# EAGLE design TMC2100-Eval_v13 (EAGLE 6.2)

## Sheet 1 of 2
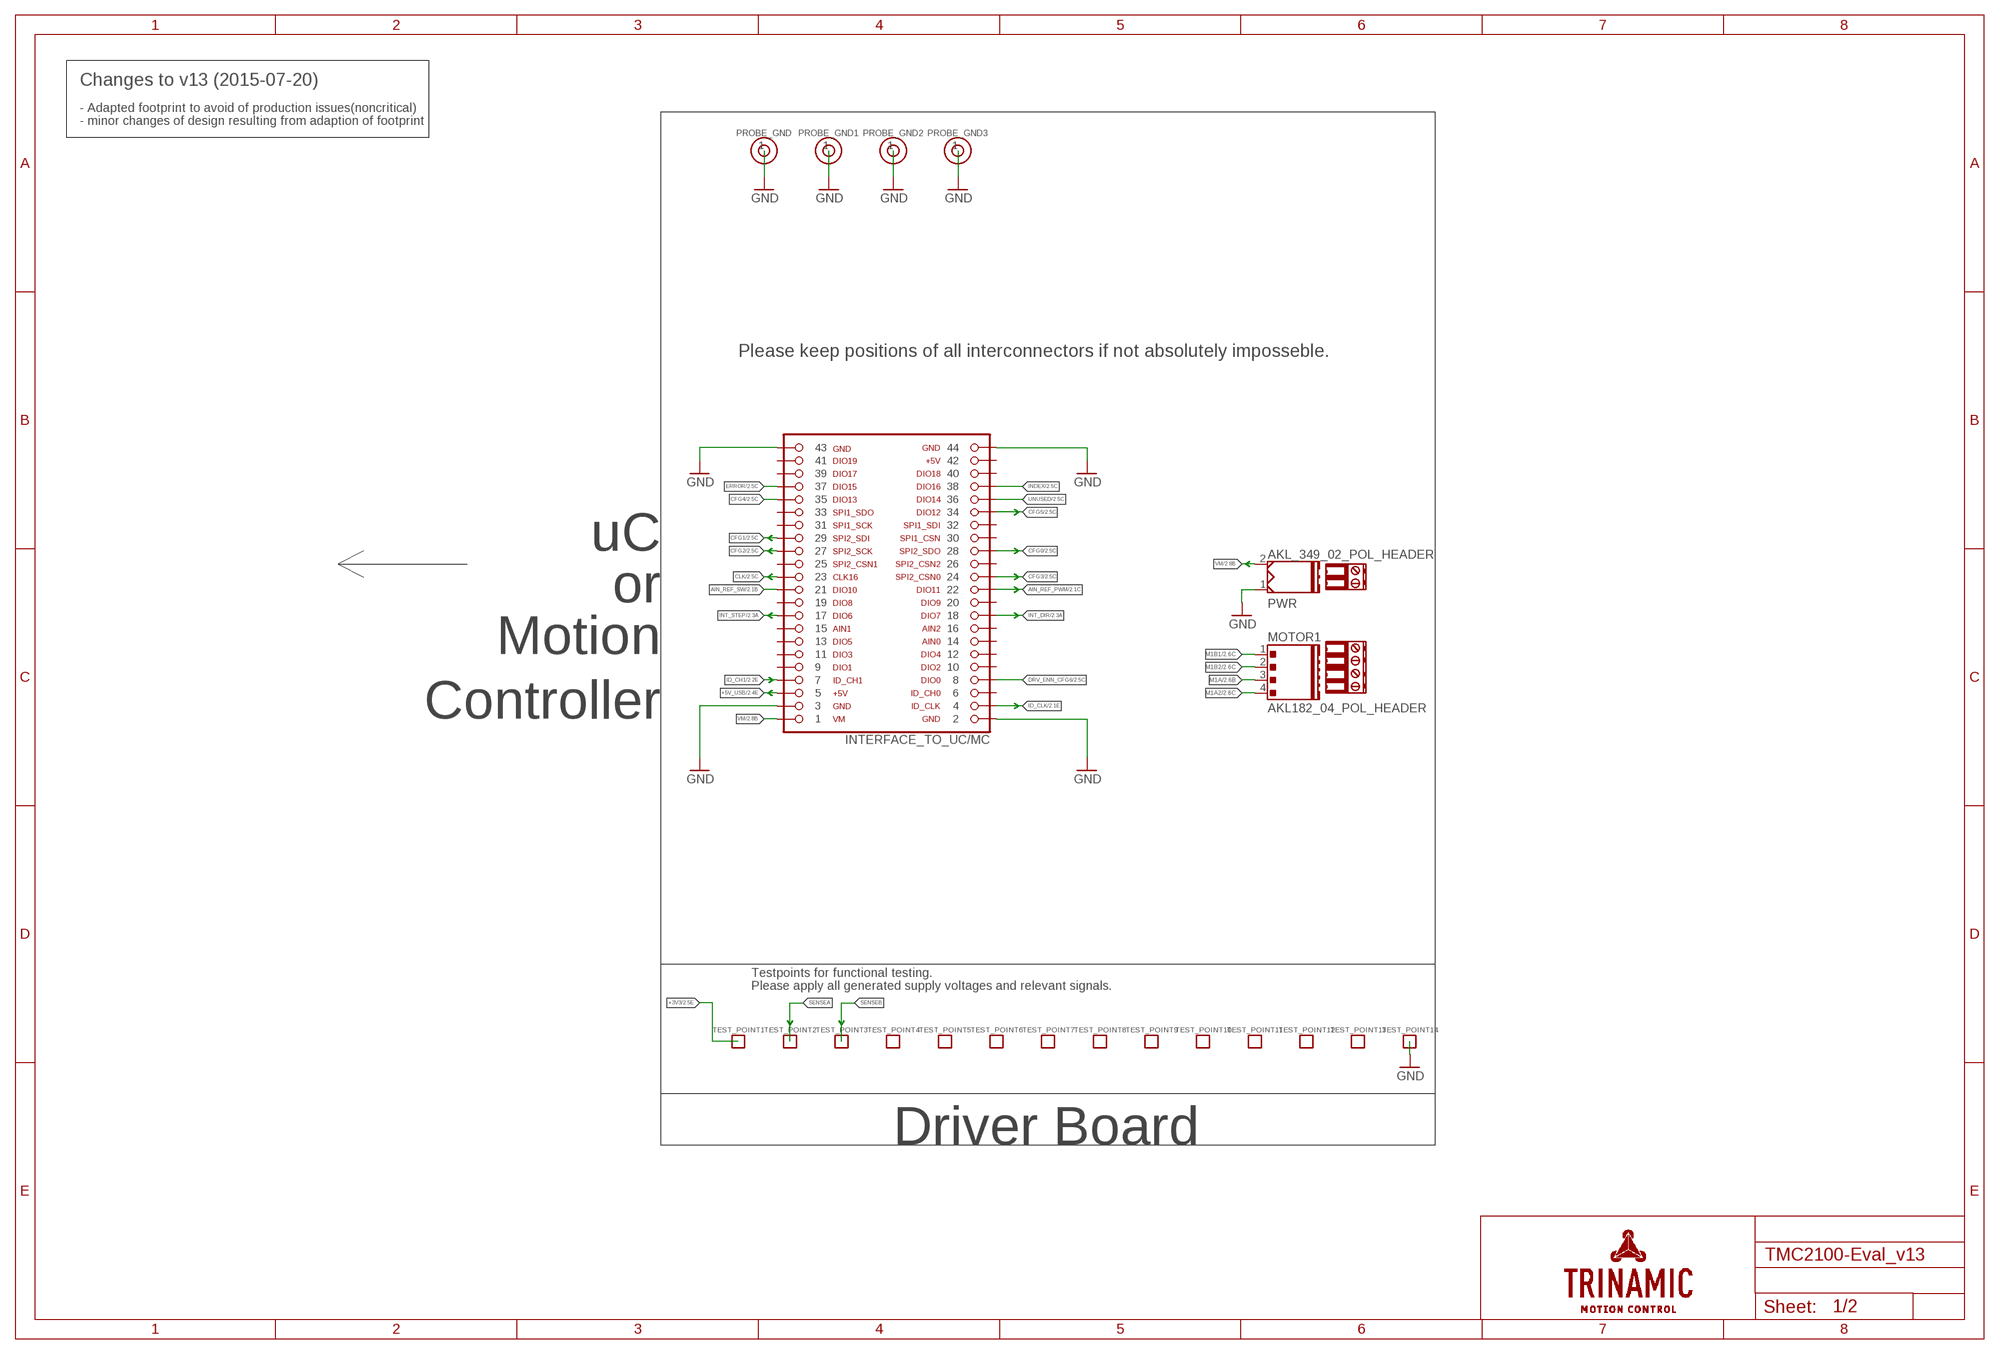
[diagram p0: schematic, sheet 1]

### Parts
INTERFACE_TO_UC/MC  FEMALE_HEADER_SMD_2.54_44_PINSHORTPADS_HOLES  [FEMALE_HEADER_SMD_254_44_PIN_SHORTPADS_HOLES]
MOTOR1  AKL182_04_POL_HEADER  [AKL169_04_POL]
PROBE_GND  NOT ASSEMBLED  1PIN_1ROW  [1PIN_1ROW_THT]
PROBE_GND1  NOT ASSEMBLED  1PIN_1ROW  [1PIN_1ROW_THT]
PROBE_GND2  NOT ASSEMBLED  1PIN_1ROW  [1PIN_1ROW_THT]
PROBE_GND3  NOT ASSEMBLED  1PIN_1ROW  [1PIN_1ROW_THT]
PWR  AKL_349_02_POL_HEADER  [AKL349_02_POL]
TERM1  AKL_330_2_POL_TERMINAL  [EXTRA_TERMINAL]
TERM2  AKL182_04_POL_TERMINAL  [EXTRA_TERMINAL]
TEST_POINT1  NOT ASSEMBLED  PAD_ROUND  [PAD_R1.2]
TEST_POINT2  NOT ASSEMBLED  PAD_ROUND  [PAD_R1.2]
TEST_POINT3  NOT ASSEMBLED  PAD_ROUND  [PAD_R1.2]
TEST_POINT4  NOT ASSEMBLED  PAD_ROUND  [PAD_R1.2]
TEST_POINT5  NOT ASSEMBLED  PAD_ROUND  [PAD_R1.2]
TEST_POINT6  NOT ASSEMBLED  PAD_ROUND  [PAD_R1.2]
TEST_POINT7  NOT ASSEMBLED  PAD_ROUND  [PAD_R1.2]
TEST_POINT8  NOT ASSEMBLED  PAD_ROUND  [PAD_R1.2]
TEST_POINT9  NOT ASSEMBLED  PAD_ROUND  [PAD_R1.2]
TEST_POINT10  NOT ASSEMBLED  PAD_ROUND  [PAD_R1.2]
TEST_POINT11  NOT ASSEMBLED  PAD_ROUND  [PAD_R1.2]
TEST_POINT12  NOT ASSEMBLED  PAD_ROUND  [PAD_R1.2]
TEST_POINT13  NOT ASSEMBLED  PAD_ROUND  [PAD_R1.2]
TEST_POINT14  NOT ASSEMBLED  PAD_ROUND  [PAD_R1.2]

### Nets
+3V3: TEST_POINT1.P$1 ; also sheet 2
+5V_USB: INTERFACE_TO_UC/MC.5 ; also sheet 2
AIN_REF_PWM: INTERFACE_TO_UC/MC.22 ; also sheet 2
AIN_REF_SW: INTERFACE_TO_UC/MC.21 ; also sheet 2
CFG0: INTERFACE_TO_UC/MC.28 ; also sheet 2
CFG1: INTERFACE_TO_UC/MC.29 ; also sheet 2
CFG2: INTERFACE_TO_UC/MC.27 ; also sheet 2
CFG3: INTERFACE_TO_UC/MC.24 ; also sheet 2
CFG4: INTERFACE_TO_UC/MC.35 ; also sheet 2
CFG5: INTERFACE_TO_UC/MC.34 ; also sheet 2
CLK: INTERFACE_TO_UC/MC.23 ; also sheet 2
DRV_ENN_CFG6: INTERFACE_TO_UC/MC.8 ; also sheet 2
ERROR: INTERFACE_TO_UC/MC.37 ; also sheet 2
GND: INTERFACE_TO_UC/MC.2 INTERFACE_TO_UC/MC.3 INTERFACE_TO_UC/MC.43 INTERFACE_TO_UC/MC.44 PROBE_GND1.1 PROBE_GND2.1 PROBE_GND3.1 PROBE_GND.1 PWR.1 TEST_POINT14.P$1 ; also sheet 2
ID_CH1: INTERFACE_TO_UC/MC.7 ; also sheet 2
ID_CLK: INTERFACE_TO_UC/MC.4 ; also sheet 2
INDEX: INTERFACE_TO_UC/MC.38 ; also sheet 2
INT_DIR: INTERFACE_TO_UC/MC.18 ; also sheet 2
INT_STEP: INTERFACE_TO_UC/MC.17 ; also sheet 2
M1A: MOTOR1.3 ; also sheet 2
M1A2: MOTOR1.4 ; also sheet 2
M1B1: MOTOR1.1 ; also sheet 2
M1B2: MOTOR1.2 ; also sheet 2
SENSEA: TEST_POINT2.P$1 ; also sheet 2
SENSEB: TEST_POINT3.P$1 ; also sheet 2
UNUSED: INTERFACE_TO_UC/MC.36 ; also sheet 2
VM: INTERFACE_TO_UC/MC.1 PWR.2 ; also sheet 2
Unconnected: INTERFACE_TO_UC/MC.6 INTERFACE_TO_UC/MC.9 INTERFACE_TO_UC/MC.10 INTERFACE_TO_UC/MC.11 INTERFACE_TO_UC/MC.12 INTERFACE_TO_UC/MC.13 INTERFACE_TO_UC/MC.14 INTERFACE_TO_UC/MC.15 INTERFACE_TO_UC/MC.16 INTERFACE_TO_UC/MC.19 INTERFACE_TO_UC/MC.20 INTERFACE_TO_UC/MC.25 INTERFACE_TO_UC/MC.26 INTERFACE_TO_UC/MC.30 INTERFACE_TO_UC/MC.31 INTERFACE_TO_UC/MC.32 INTERFACE_TO_UC/MC.33 INTERFACE_TO_UC/MC.39 INTERFACE_TO_UC/MC.40 INTERFACE_TO_UC/MC.41 INTERFACE_TO_UC/MC.42 TEST_POINT4.P$1 TEST_POINT5.P$1 TEST_POINT6.P$1 TEST_POINT7.P$1 TEST_POINT8.P$1 TEST_POINT9.P$1 TEST_POINT10.P$1 TEST_POINT11.P$1 TEST_POINT12.P$1 TEST_POINT13.P$1

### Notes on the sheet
- Changes to v13 (2015-07-20)
- - Adapted footprint to avoid of production issues(noncritical)
- - minor changes of design resulting from adaption of footprint
- Please keep positions of all interconnectors if not absolutely imposseble.
- uC
- or
- Motion
- Controller
- Testpoints for functional testing.
- Please apply all generated supply voltages and relevant signals.
- Driver Board

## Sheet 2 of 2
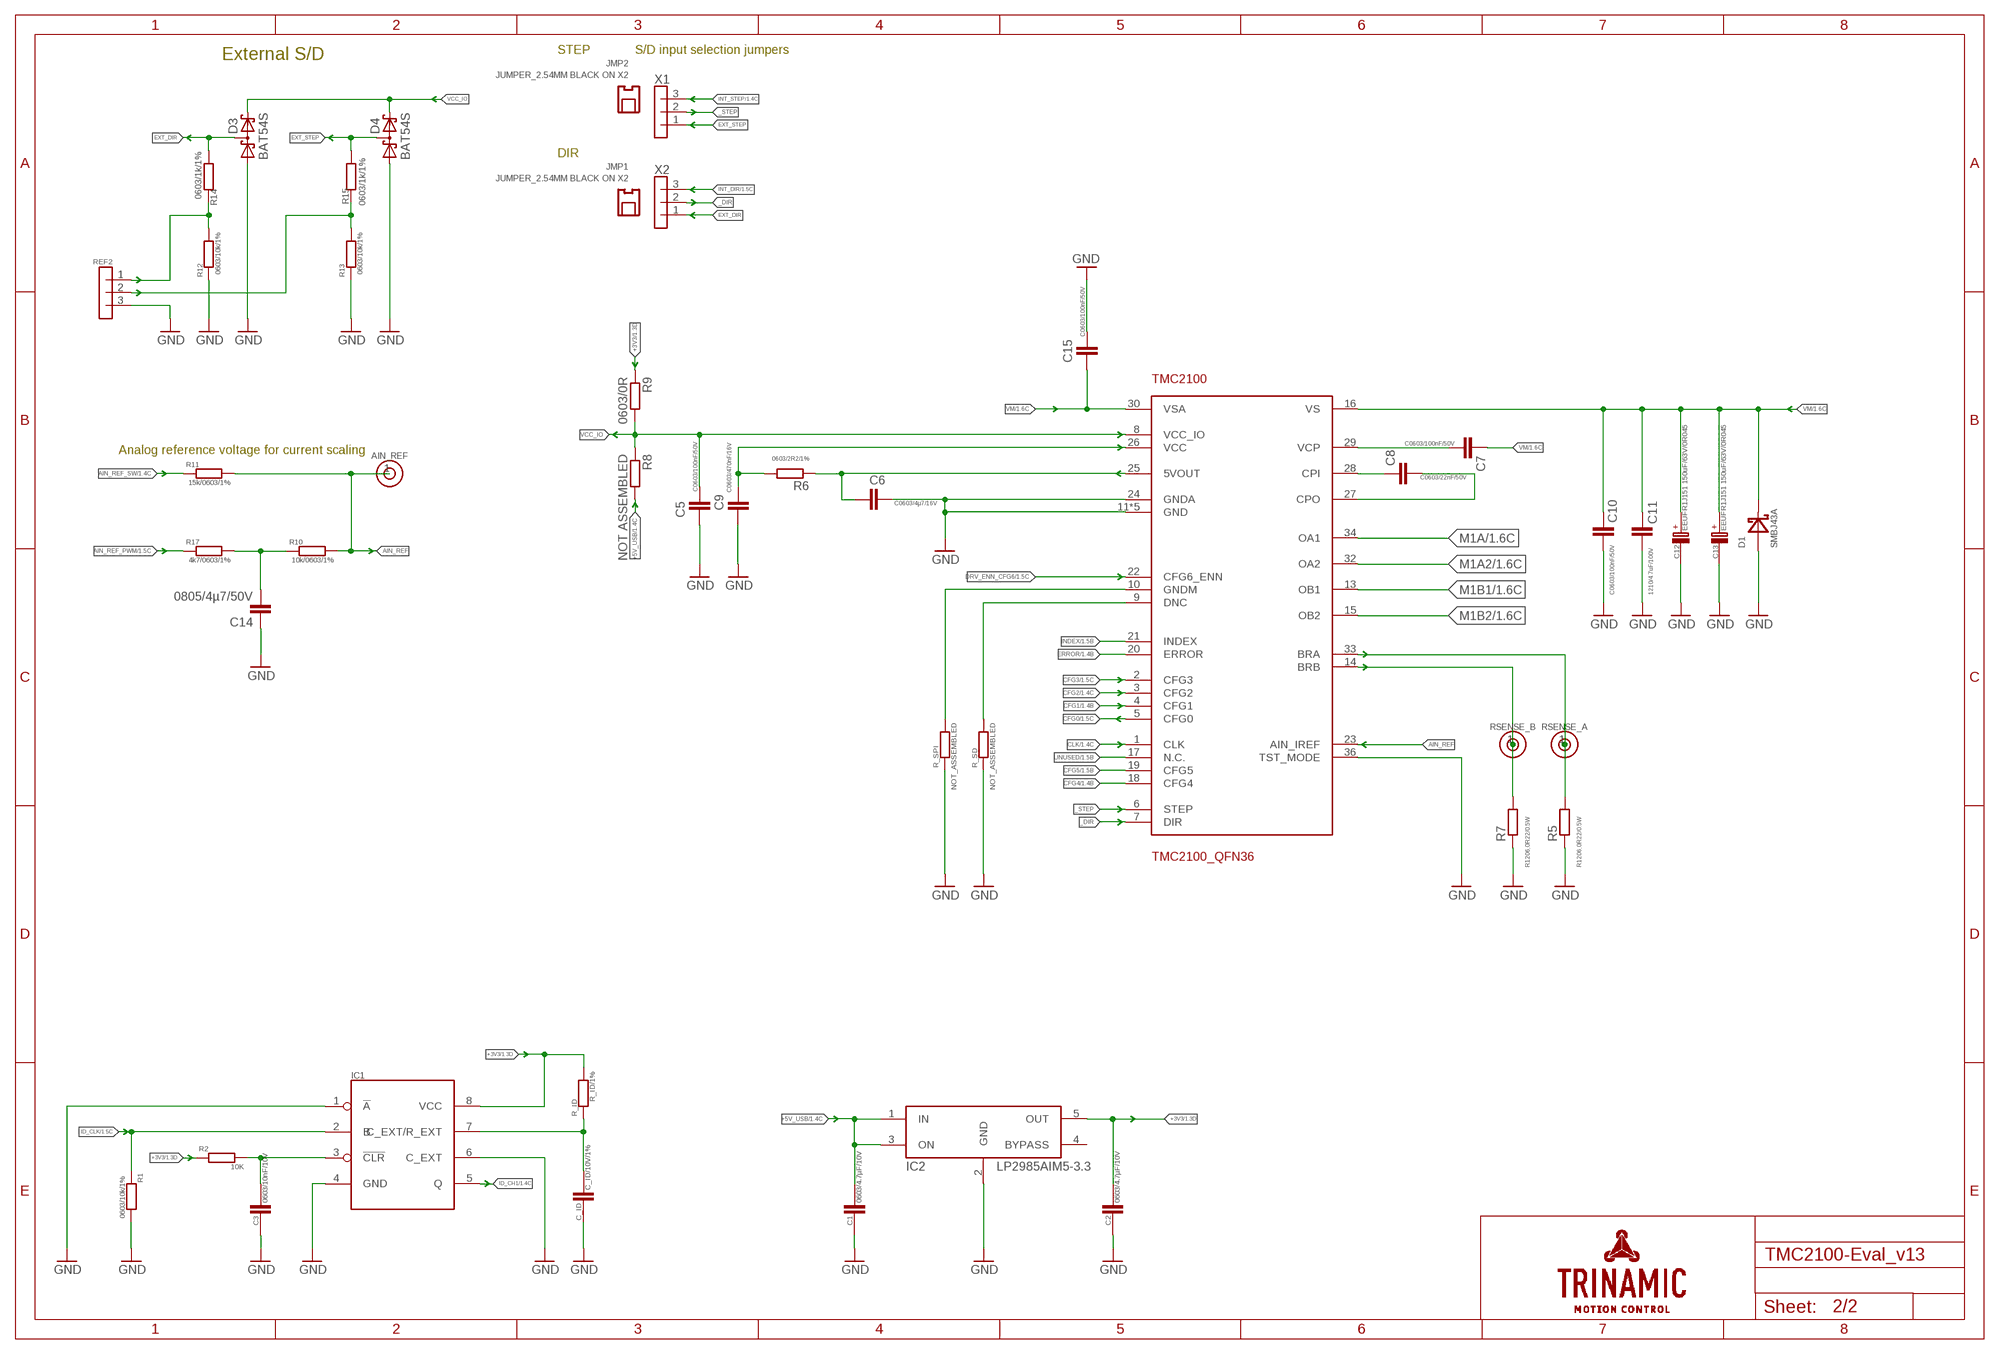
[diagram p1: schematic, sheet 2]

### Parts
AIN_REF  NOT ASSEMBLED  1PIN_1ROW  [1PIN_1ROW_THT]
C1  0603/4.7µF/10V  RCL_C/0603  [RCL_0603]
C2  0603/4.7µF/10V  RCL_C/0603  [RCL_0603]
C3  0603/10nF/10V  RCL_C/0603  [RCL_0603]
C5  C0603/100nF/50V  C-EUC0603  [C0603]
C6  C0603/4µ7/16V  C-EUC0603  [C0603]
C7  C0603/100nF/50V  C-EUC0603  [C0603]
C8  C0603/22nF/50V  C-EUC0603  [C0603]
C9  C0603/470nF/16V  C-EUC0603  [C0603]
C10  C0603/100nF/50V  C-EUC0603  [C0603]
C11  1210/4.7uF/100V  C-EUC1210  [C1210]
C12  EEUFR1J151 150uF/63V/0R045  C_POL  [C_POL_RAD_THT_5X10X12.5]
C13  EEUFR1J151 150uF/63V/0R045  C_POL  [C_POL_RAD_THT_5X10X12.5]
C14  0805/4µ7/50V  C-EUC0805  [C0805]
C15  C0603/100nF/50V  C-EUC0603  [C0603]
C_ID  C_ID/10V/1%  RCL_C/0603  [RCL_0603]
D1  SMBJ43A  SMBJ  [SMB]
D3  BAT54S  [SOT23]
D4  BAT54S  [SOT23]
IC1  SN74LVC1G123DCTR  [SN74LVC1G123DCTR]
IC2  LP2985AIM5-3.3  [SOT23-5]
JMP1  JUMPER_2.54MM BLACK ON X2  JUMPER_2.54MM  [EXTRA_TERMINAL]
JMP2  JUMPER_2.54MM BLACK ON X2  JUMPER_2.54MM  [EXTRA_TERMINAL]
R1  0603/10k/1%  RCL_R/0603  [RCL_0603]
R2  10K  RCL_R/0603  [RCL_0603]
R5  R1206,0R22/0.5W  R-EU_R1206  [R1206]
R6  0603/2R2/1%  R-EU_R0603  [R0603]
R7  R1206,0R22/0.5W  R-EU_R1206  [R1206]
R8  NOT ASSEMBLED  R-EU_R0603  [R0603]
R9  0603/0R  R-EU_R0603  [R0603]
R10  10k/0603/1%  RCL_R/0603  [RCL_0603]
R11  15k/0603/1%  RCL_R/0603  [RCL_0603]
R12  0603/10k/1%  R/0603  [0603]
R13  0603/10k/1%  R/0603  [0603]
R14  0603/1k/1%  R/0603  [0603]
R15  0603/1k/1%  R/0603  [0603]
R17  4k7/0603/1%  RCL_R/0603  [RCL_0603]
R_ID  R_ID/1%  RCL_R/0603  [RCL_0603]
R_SD  NOT_ASSEMBLED  RCL_R/0603  [RCL_0603]
R_SPI  NOT_ASSEMBLED  RCL_R/0603  [RCL_0603]
REF2  MALE HEADER 2.54  3PIN_1ROWTHT  [3PIN_1ROW_2,54_THT]
RSENSE_A  NOT ASSEMBLED  1PIN_1ROW  [1PIN_1ROW_THT]
RSENSE_B  NOT ASSEMBLED  1PIN_1ROW  [1PIN_1ROW_THT]
TMC2100  TMC2100_QFN36  [QFN36]
X1  MALE HEADER 2.54  3PIN_1ROWTHT  [3PIN_1ROW_2,54_THT]
X2  MALE HEADER 2.54  3PIN_1ROWTHT  [3PIN_1ROW_2,54_THT]

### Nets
+3V3: C2.1 IC1.8(VCC) IC2.5(OUT) R2.1 R9.1 R_ID.2 ; also sheet 1
+5V_USB: C1.1 IC2.1(IN) IC2.3(ON) R8.2 ; also sheet 1
_DIR: TMC2100.7(DIR) X2.2
_STEP: TMC2100.6(STEP) X1.2
AIN_REF: AIN_REF.1 R10.2 R11.2 TMC2100.23(AIN_IREF)
AIN_REF_PWM: R17.1 ; also sheet 1
AIN_REF_SW: R11.1 ; also sheet 1
CFG0: TMC2100.5(CFG0) ; also sheet 1
CFG1: TMC2100.4(CFG1) ; also sheet 1
CFG2: TMC2100.3(CFG2) ; also sheet 1
CFG3: TMC2100.2(CFG3) ; also sheet 1
CFG4: TMC2100.18(CFG4) ; also sheet 1
CFG5: TMC2100.19(CFG5) ; also sheet 1
CLK: TMC2100.1(CLK) ; also sheet 1
DRV_ENN_CFG6: TMC2100.22(CFG6_ENN) ; also sheet 1
ERROR: TMC2100.20(ERROR) ; also sheet 1
EXT_DIR: D3.3(C1A2) R14.2 X2.1
EXT_DIR_CON: R12.2 R14.1 REF2.1
EXT_STEP: D4.3(C1A2) R15.2 X1.1
EXT_STEP_CON: R13.2 R15.1 REF2.2
GND: C1.2 C2.2 C3.2 C5.2 C6.2 C9.1 C10.1 C11.2 C12.- C13.- C14.1 C15.1 C_ID.2 D1.A D3.1(A1) D4.1(A1) IC1.1(!A) IC1.4(GND) IC1.6(C_EXT) IC2.2(GND) R1.2 R5.1 R7.1 R12.1 R13.1 R_SD.1 R_SPI.1 REF2.3 TMC2100.11(GND) TMC2100.12(GND) TMC2100.24(GNDA) TMC2100.31(GND) TMC2100.35(GND) TMC2100.36(TST_MODE) TMC2100.GND_PAD(GND) ; also sheet 1
ID_CH1: IC1.5(Q) ; also sheet 1
ID_CLK: IC1.2(B) R1.1 ; also sheet 1
INDEX: TMC2100.21(INDEX) ; also sheet 1
INT_DIR: X2.3 ; also sheet 1
INT_STEP: X1.3 ; also sheet 1
M1A: TMC2100.34(OA1) ; also sheet 1
M1A2: TMC2100.32(OA2) ; also sheet 1
M1B1: TMC2100.13(OB1) ; also sheet 1
M1B2: TMC2100.15(OB2) ; also sheet 1
N$1: C3.1 IC1.3(!CLR) R2.2
N$2: C_ID.1 IC1.7(C_EXT/R_EXT) R_ID.1
N$3: R_SPI.2 TMC2100.10(GNDM)
N$5: R_SD.2 TMC2100.9(DNC)
N$7: C6.1 R6.1 TMC2100.25(5VOUT)
N$8: C8.1 TMC2100.28(CPI)
N$9: C8.2 TMC2100.27(CPO)
N$10: C7.2 TMC2100.29(VCP)
N$11: C9.2 R6.2 TMC2100.26(VCC)
N$14: C14.2 R10.1 R17.2
SENSEA: R5.2 RSENSE_A.1 TMC2100.33(BRA) ; also sheet 1
SENSEB: R7.2 RSENSE_B.1 TMC2100.14(BRB) ; also sheet 1
UNUSED: TMC2100.17(N.C.) ; also sheet 1
VCC_IO: C5.1 D3.2(C2) D4.2(C2) R8.1 R9.2 TMC2100.8(VCC_IO)
VM: C7.1 C10.2 C11.1 C12.+ C13.+ C15.2 D1.C TMC2100.16(VS) TMC2100.30(VSA) ; also sheet 1
Unconnected: IC2.4(BYPASS)

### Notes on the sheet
- STEP | S/D input selection jumpers
- External S/D
- DIR
- Analog reference voltage for current scaling

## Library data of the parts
AIN_REF PROBE_GND PROBE_GND1-PROBE_GND3 RSENSE_A RSENSE_B = _TMC_TE_con:1PIN_1ROW
C1-C3 C_ID = TMC_EVAL_driver_TE_v01:RCL_C
C5-C11 C14 C15 = rcl:C-EU: CAPACITOR, European symbol
C12 C13 = _TMC_TE_RCL:C_POL
D1 = _TMC_TE_D:SMBJ
D3 D4 = Trinamic:BAT54S: SOT23, BAT54S, Double Schottky diode 30V 200mA Copied from diode.lbr and edited for Artec use 23-08-13 Pin connection corrected 2011-05-04 Source: Fairchild .. BAT54.pdf; ADGPN: 3522154300; DATASHEET: http://www.nxp.com/documents/data_sheet/BAT54_SERIES.pdf; MANUF-CODE-1: BAT54S; MANUFACTURER-1: Philips; PRICE: 0.11
IC1 = TMC_EVAL_driver_TE_v01:SN74LVC1G123DCTR
IC2 = TMC_EVAL_driver_TE_v01:LP2985AIM5-3.3
INTERFACE_TO_UC/MC = _TMC_TE_con:FEMALE_HEADER_SMD_2.54_44_PIN; 1_PARTNUMBER: 098-3-044-1-NFX-YT0; 1_SUPPLIER: MPE Garry; 2_PARTNUMBER: HLE-122-02-F-DV-A; 2_SUPPLIER: Samtec
JMP1 JMP2 = _TMC_TE_con:JUMPER_2.54MM: Jumper 2.54mm, Open top, h6.5mm, black
MOTOR1 = _TMC_TE_con:AKL182_04_POL_HEADER: AKL header, shrouted, 4 pins; 1_PARTNUMBER: 31182104; 1_SUPPLIER: RIA CONNECT; 2_PARTNUMBER: AKL 182-04; 2_SUPPLIER: Reichelt
PWR = _TMC_TE_con:AKL_349_02_POL_HEADER: AKL header, shrouted, 2 pins; 1_PARTNUMBER: 31330102; 1_SUPPLIER: RIA CONNECT; 2_PARTNUMBER: AKL 330-02; 2_SUPPLIER: REICHELT
R1 R2 R10 R11 R17 R_ID R_SD R_SPI = TMC_EVAL_driver_TE_v01:RCL_R
R5-R9 = rcl:R-EU_: RESISTOR, European symbol
R12-R15 = _TMC_TE_RCL:R
REF2 X1 X2 = _TMC_TE_con:3PIN_1ROW
TERM1 = _TMC_TE_con:AKL_330_2_POL_TERMINAL: AKL terminal, 2 pins; 1_PARTNUMBER: 31349102; 1_SUPPLIER: RIA CONNECT; 2_PARTNUMBER: AKL 349-02; 2_SUPPLIER: Reichelt
TERM2 = _TMC_TE_con:AKL182_04_POL_TERMINAL: AKL terminal, 4 pins; 1_PARTNUMBER: 31169104; 1_SUPPLIER: RIA CONNECT; 2_PARTNUMBER: AKL 169-04; 2_SUPPLIER: Reichelt
TEST_POINT1-TEST_POINT14 = _TMC_TE_PADS:PAD_ROUND
TMC2100 = Trinamic:TMC2100_QFN36

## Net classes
0 default: width 0.254 mm, drill 0.3 mm

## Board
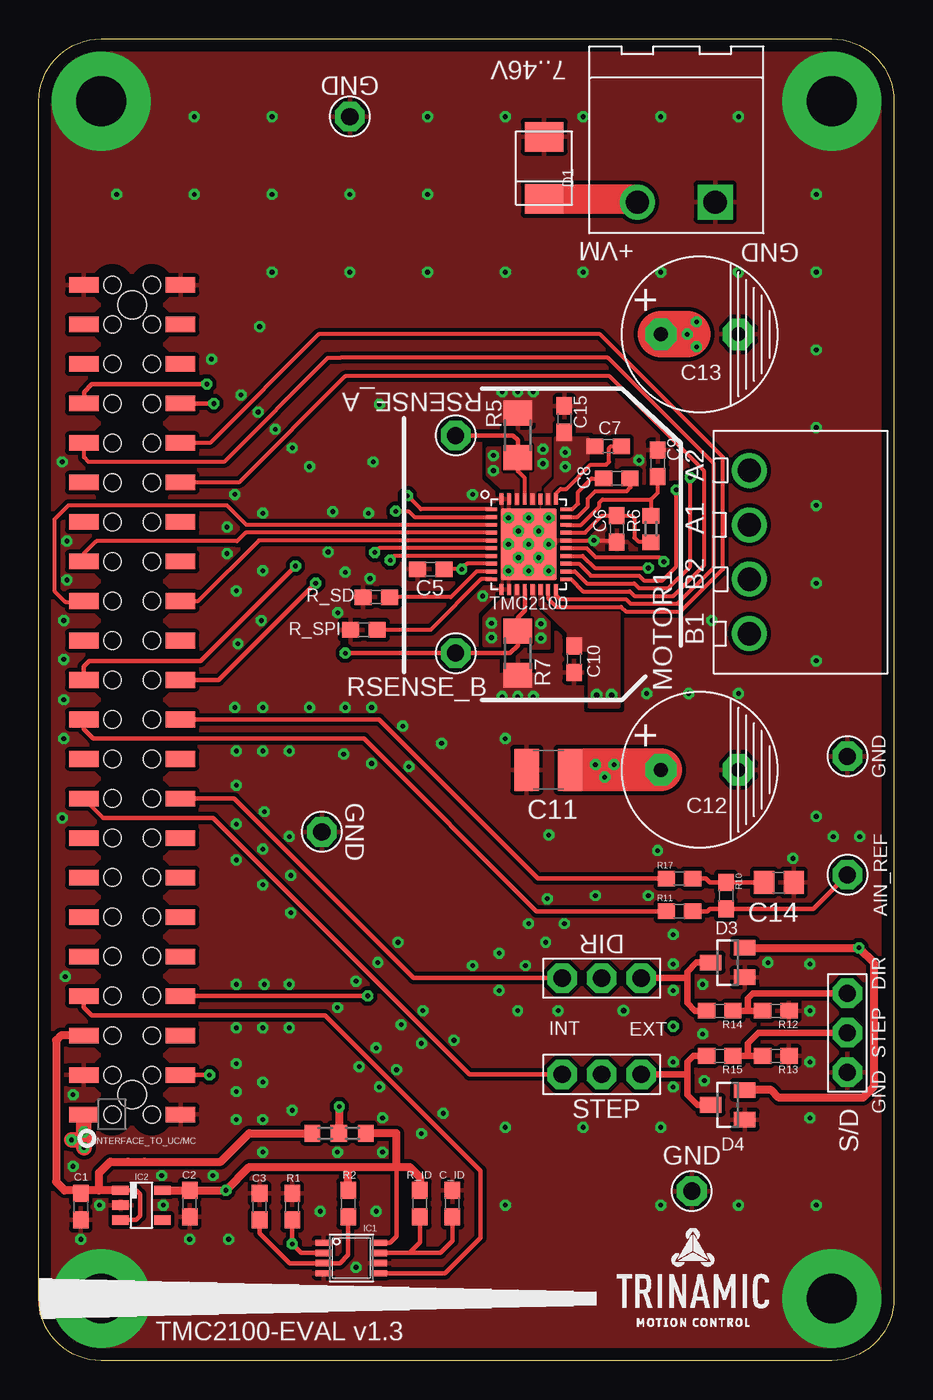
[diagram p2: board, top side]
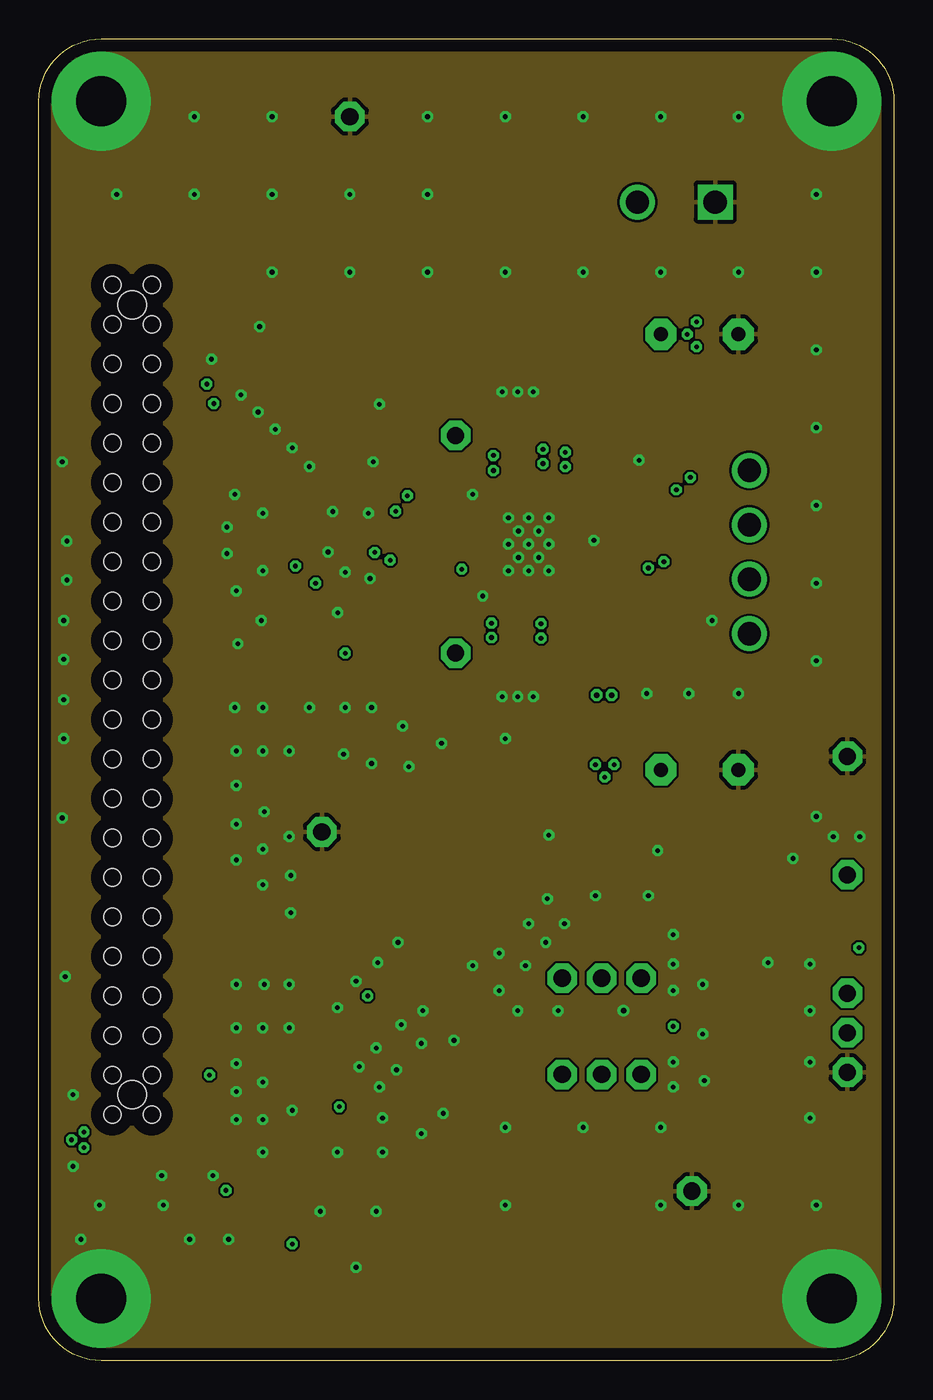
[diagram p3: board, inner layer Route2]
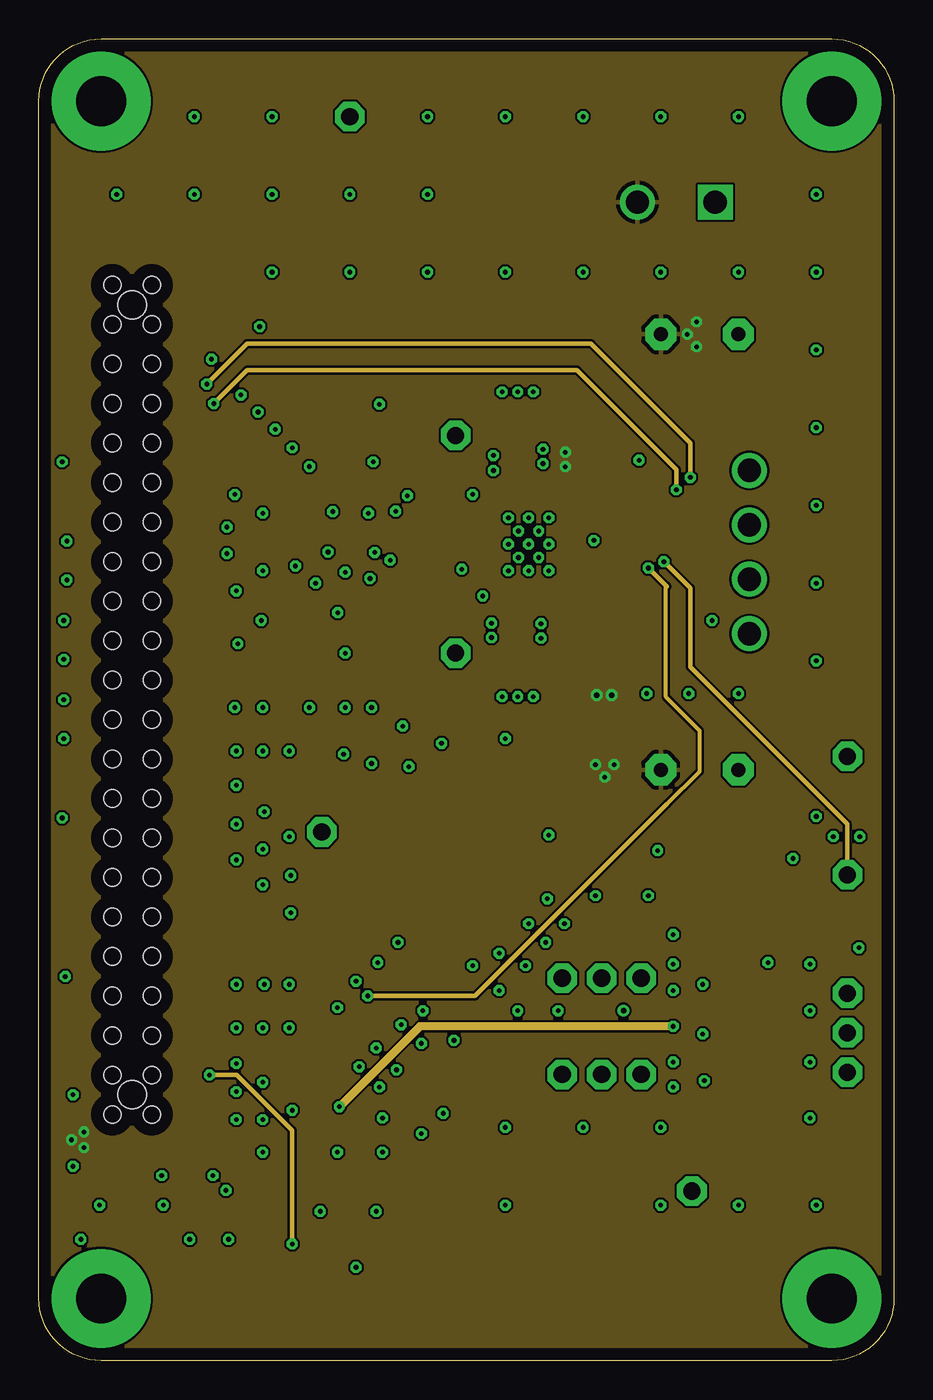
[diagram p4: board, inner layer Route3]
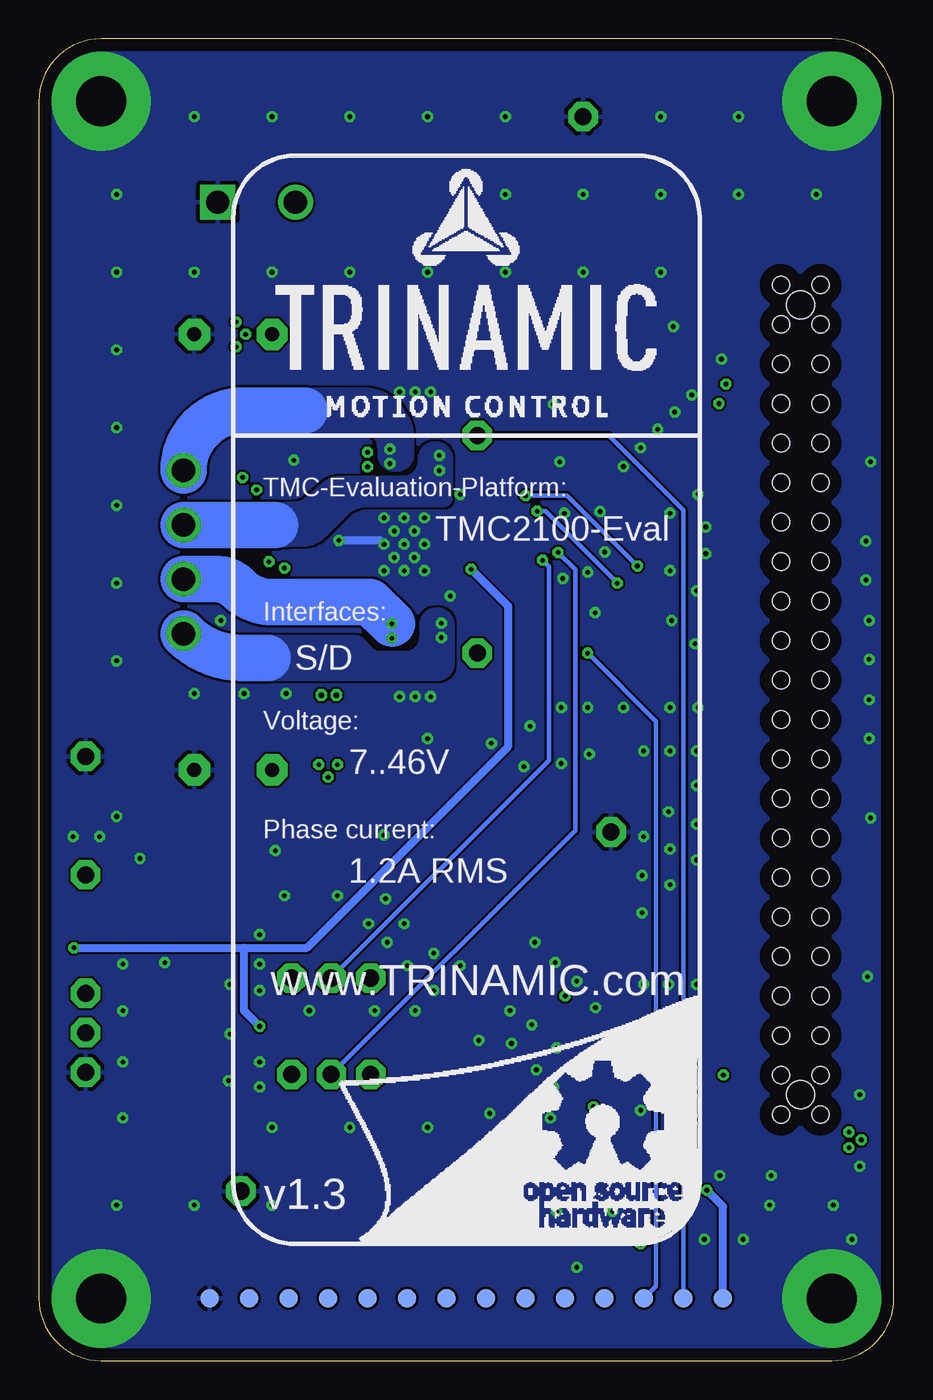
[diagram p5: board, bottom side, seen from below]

Size 55 x 85 mm. Coordinates in mm from the lower left corner, seen from the top.
Outline: 51,0 4,0 arc-90 0,4 0,81 arc-90 4,85 51,85 arc-90 55,81 55,4 arc-90 51,0
Copper layers (1*2*3*16): Top 0.018mm / dielectric 0.36mm / Route2 0.035mm / dielectric 0.71mm / Route3 0.035mm / dielectric 0.2mm / Bottom 0.018mm
Design rules: minimum track width 0.15mm, minimum drill 0.25mm, track to track 0.15mm, track to pad 0.15mm, pad to pad 0.1mm, via to via 0.15mm, smd to smd 0mil, copper to edge 0.8mm, drill to drill 8mil, minimum pad ring 10mil, minimum via ring 8mil, stop-mask expansion 4mil, vias tented up to drill 0.4mm, thermal gap 10mil

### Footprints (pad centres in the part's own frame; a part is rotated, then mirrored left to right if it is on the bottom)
1PIN_1ROW_THT = drill 1.1 pad 1.9 octagon: 1 0,0
RCL_0603 = smd 1.1 x 1: 1 -0.85,0; 2 0.85,0
C0603 = smd 1.1 x 1: 1 -0.85,0; 2 0.85,0
C1210 = smd 1.6 x 2.7: 1 -1.4,0; 2 1.4,0
C_POL_RAD_THT_5X10X12.5 = drill 0.9 pad 2 octagon: + 2.5,0; - -2.5,0
C0805 = smd 1.3 x 1.5: 1 -0.95,0; 2 0.95,0
SMB = smd 1.9 x 2.5: A 2,0; C -2,0
SOT23 = smd 1 x 1.4: 1 -0.95,-1.1; 2 0.95,-1.1; 3 0,1.1
SN74LVC1G123DCTR = smd 0.4 x 1: 1 -0.975,-1.8; 2 -0.325,-1.8; 3 0.325,-1.8; 4 0.975,-1.8; 5 0.975,1.8; 6 0.325,1.8; 7 -0.325,1.8; 8 -0.975,1.8
SOT23-5 = smd 0.6 x 1.05: 1 -0.95,-1.35; 2 0,-1.35; 3 0.95,-1.35; 4 0.95,1.35; 5 -0.95,1.35
FEMALE_HEADER_SMD_254_44_PIN_SHORTPADS_HOLES = smd 1 x 1.9: 1 -26.67,3.11; 2 -26.67,-3.11; 3 -24.13,3.11; 4 -24.13,-3.11; 5 -21.59,3.11; 6 -21.59,-3.11; 7 -19.05,3.11; 8 -19.05,-3.11; 9 -16.51,3.11; 10 -16.51,-3.11; 11 -13.97,3.11; 12 -13.97,-3.11; 13 -11.43,3.11; 14 -11.43,-3.11; 15 -8.89,3.11; 16 -8.89,-3.11; 17 -6.35,3.11; 18 -6.35,-3.11; 19 -3.81,3.11; 20 -3.81,-3.11; 21 -1.27,3.11; 22 -1.27,-3.11; 23 1.27,3.11; 24 1.27,-3.11; 25 3.81,3.11; 26 3.81,-3.11; 27 6.35,3.11; 28 6.35,-3.11; 29 8.89,3.11; 30 8.89,-3.11; 31 11.43,3.11; 32 11.43,-3.11; 33 13.97,3.11; 34 13.97,-3.11; 35 16.51,3.11; 36 16.51,-3.11; 37 19.05,3.11; 38 19.05,-3.11; 39 21.59,3.11; 40 21.59,-3.11; 41 24.13,3.11; 42 24.13,-3.11; 43 26.67,3.11; 44 26.67,-3.11 | hole 1.8: -25.4,0; 25.4,0 | hole 1.1: -26.67,1.27; -24.13,1.27; -21.59,1.27; -19.05,1.27; -16.51,1.27; -13.97,1.27; -11.43,1.27; -8.89,1.27; -6.35,1.27; -3.81,1.27; -1.27,1.27; 1.27,1.27; 3.81,1.27; 6.35,1.27; 8.89,1.27; 11.43,1.27; 13.97,1.27; 16.51,1.27; 19.05,1.27; 21.59,1.27; 24.13,1.27; 26.67,1.27; -26.67,-1.27; -24.13,-1.27; -21.59,-1.27; -19.05,-1.27; -16.51,-1.27; -13.97,-1.27; -11.43,-1.27; -8.89,-1.27; -6.35,-1.27; -3.81,-1.27; -1.27,-1.27; 1.27,-1.27; 3.81,-1.27; 6.35,-1.27; 8.89,-1.27; 11.43,-1.27; 13.97,-1.27; 16.51,-1.27; 19.05,-1.27; 21.59,-1.27; 24.13,-1.27; 26.67,-1.27
AKL169_04_POL = drill 1.5: 1 -5.25,3.3; 2 -1.75,3.3; 3 1.75,3.3; 4 5.25,3.3
AKL349_02_POL = drill 1.5 square: 1 -2.5,4 | drill 1.5: 2 2.5,4
R1206 = smd 1.6 x 1.803: 1 -1.422,0; 2 1.422,0
R0603 = smd 1 x 1.1: 1 -0.85,0; 2 0.85,0
0603 = smd 1.1 x 1: 1 -0.85,0; 2 0.85,0
3PIN_1ROW_2,54_THT = drill 1.1 pad 1.9 octagon: 1 -2.54,0; 2 0,0; 3 2.54,0
PAD_R1.2 = smd 1.2 x 1.2: P$1 0,0
QFN36 = smd 0.7 x 0.25: 1 -2.4,2.25; 2 -2.4,1.75; 3 -2.4,1.25; 4 -2.4,0.75; 5 -2.4,0.25; 6 -2.4,-0.25; 7 -2.4,-0.75; 8 -2.4,-1.25; 9 -2.4,-1.75; 10 -2.4,-2.25; 19 2.4,-2.25; 20 2.4,-1.75; 21 2.4,-1.25; 22 2.4,-0.75; 23 2.4,-0.25; 24 2.4,0.25; 25 2.4,0.75; 26 2.4,1.25; 27 2.4,1.75; 28 2.4,2.25 | smd 0.25 x 0.7: 11 -1.75,-2.9; 12 -1.25,-2.9; 13 -0.75,-2.9; 14 -0.25,-2.9; 15 0.25,-2.9; 16 0.75,-2.9; 17 1.25,-2.9; 18 1.75,-2.9; 29 1.75,2.9; 30 1.25,2.9; 31 0.75,2.9; 32 0.25,2.9; 33 -0.25,2.9; 34 -0.75,2.9; 35 -1.25,2.9; 36 -1.75,2.9 | smd 3.6 x 4.6: GND_PAD 0,0

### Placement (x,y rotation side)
AIN_REF  52,31.24 90 top
C1  2.7,9.9 270 top
C2  9.7,10.1 270 top
C3  14.2,9.9 90 top
C5  25.2,50.9 180 top
C6  37.17,53.49 270 top
C7  36.61,58.8 0 top
C8  37.17,56.74 0 top
C9  39.8,57.7 270 top
C10  34.42,45.11 90 top
C11  32.77,38 180 top
C12  42.5,38 180 top
C13  42.5,66 180 top
C14  47.6,30.75 180 top
C15  33.8,60.55 270 top
C_ID  26.6,10.1 90 top
D1  32.5,76.7 90 top
D3  44.3,25.6 90 top
D4  44.3,16.45 90 top
IC1  20.1,6.6 270 top
IC2  6.6,10 270 top
INTERFACE_TO_UC/MC  6,42.5 90 top
JMP1  not placed on the board
JMP2  not placed on the board
MOTOR1  49,52 90 top
PROBE_GND  18.2,34 0 top
PROBE_GND1  52,38.86 180 top
PROBE_GND2  42,10.9 0 top
PROBE_GND3  20,80 180 top
PWR  41,78.5 180 top
R1  16.3,9.9 90 top
R2  19.9,10.1 270 top
R5  30.8,59.5 270 top
R6  39.36,53.49 90 top
R7  30.8,45.5 90 top
R8  18.43,14.62 180 top
R9  20.18,14.62 180 top
R10  44.2,29.9 270 top
R11  41.2,28.9 0 top
R12  47.4,22.5 180 top
R13  47.4,19.6 180 top
R14  43.8,22.5 180 top
R15  43.8,19.6 180 top
R17  41.2,31 0 top
R_ID  24.5,10.1 90 top
R_SD  21.7,49.1 0 top
R_SPI  20.9,47 0 top
REF2  52,21.08 270 top
RSENSE_A  26.8,59.5 0 top
RSENSE_B  26.8,45.5 0 top
TERM1  -1,-2 0 top
TERM2  not placed on the board
TEST_POINT1  11,4 0 bottom
TEST_POINT2  13.54,4 0 bottom
TEST_POINT3  16.08,4 0 bottom
TEST_POINT4  18.62,4 0 bottom
TEST_POINT5  21.16,4 0 bottom
TEST_POINT6  26.24,4 0 bottom
TEST_POINT7  23.7,4 0 bottom
TEST_POINT8  28.78,4 0 bottom
TEST_POINT9  31.32,4 0 bottom
TEST_POINT10  33.86,4 0 bottom
TEST_POINT11  36.4,4 0 bottom
TEST_POINT12  38.94,4 0 bottom
TEST_POINT13  41.48,4 0 bottom
TEST_POINT14  44.02,4 0 bottom
TMC2100  31.5,52.5 0 top
U$1  [TMC_EVAL_RIGHT_BAR]  0,0 0 top
U$3  [TMC_EVAL_BACK_NO_DOCU]  55,0 0 bottom
X1  36.2,18.4 180 top
X2  36.2,24.6 180 top

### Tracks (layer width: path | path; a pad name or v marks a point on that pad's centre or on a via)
+3V3  (via drill 0.3)
  Top 0.3: IC1.8 22.57,7.58 23,8 23,12.45
  Top 0.406: 21.05,14.6 R9.1
  Top 0.5: IC2.5 C2.1 v12.03,10.95 13.53,12.45 19.9,12.45 | 19.9,12.45 22.7,12.45 23,12.45 | 23,12.45 23.85,12.45 24.5,11.8 R_ID.2 | R2.1 19.9,12.45 | 23,12.45 23,14.62 R9.1
  Bottom 0.5: TEST_POINT1.P$1 11,9.92 v12.03,10.95
+5V_USB
  Top 0.3: IC2.1 6.25,10.95 6.5,10.7 6.5,9.3 6.25,9.05 IC2.3
  Top 0.5: IC2.1 3.88,10.95 | 3.88,10.95 2.5,10.95 | 2.5,10.95 C1.1 | 2.51,20.91 INTERFACE_TO_UC/MC.5 1.41,20.91 1.1,20.6 1.1,11.5 1.65,10.95 2.5,10.95 | R8.2 13.53,14.62 11.7,12.8 6.8,12.8 5.73,12.8 4.6,12.8 3.88,12.08 3.88,10.95
_DIR  (via drill 0.3)
  Top 0.254: TMC2100.7 22.88,51.75 v22.6,51.48
  Bottom 0.3: X2.2 22.2,38.6 22.2,51.08 v22.6,51.48
_STEP  (via drill 0.3)
  Top 0.254: TMC2100.6 21.88,52.25 v21.6,51.98
  Bottom 0.3: X1.2 20.5,34.1 20.5,50.88 v21.6,51.98
AIN_REF  (via drill 0.3)
  Top 0.254: TMC2100.23 35.23,52.25 35.8,51.67 39.9,51.67 v40.2,51.38
  Top 0.3: R11.2 43,28.9 43.15,29.05 R10.2 49.81,29.05 AIN_REF.1
  Route3 0.3: AIN_REF.1 52,34.5 41.9,44.6 41.9,49.67 v40.2,51.38
AIN_REF_PWM
  Top 0.3: INTERFACE_TO_UC/MC.22 21.87,41.23 32.1,31 R17.1
AIN_REF_SW
  Top 0.3: INTERFACE_TO_UC/MC.21 2.89,40.61 3.5,40 20.9,40 32,28.9 R11.1
CFG0
  Top 0.254: INTERFACE_TO_UC/MC.28 10.25,48.85 14.15,52.75 TMC2100.5
CFG1
  Top 0.254: INTERFACE_TO_UC/MC.29 2.89,51.89 3.7,52.7 12.75,52.7 13.3,53.25 TMC2100.4
CFG2
  Top 0.254: INTERFACE_TO_UC/MC.27 2.84,48.8 1.7,48.8 1,49.5 1,54.1 1.9,55 12.1,55 13.35,53.75 TMC2100.3
CFG3  (via drill 0.3)
  Top 0.254: v22.95,54.62 23.77,54.62 24.15,54.25 TMC2100.2
  Top 0.3: INTERFACE_TO_UC/MC.24 11.57,43.77 v17.8,50
  Bottom 0.254: 22.52,54.62 v22.95,54.62
  Bottom 0.3: v17.8,50 22.43,54.62 v22.95,54.62
CFG4
  Top 0.254: TMC2100.18 33.25,49.23 33.5,48.98 37.75,48.98 38.05,48.67 41.08,48.67 43.4,51 43.4,57.7 36.6,64.5 19.4,64.5 18.6,64.5 11.9,57.8 3.2,57.8 2.9,58.1 INTERFACE_TO_UC/MC.35
CFG5
  Top 0.254: TMC2100.19 34.23,50.25 35,49.48 38,49.48 38.3,49.17 40.8,49.17 42.8,51.17 42.8,57.2 36.7,63.3 19.7,63.3 12.87,56.47 INTERFACE_TO_UC/MC.34
CLK  (via drill 0.3)
  Top 0.254: TMC2100.1 24.57,54.75 v23.7,55.62
  Top 0.3: INTERFACE_TO_UC/MC.23 2.89,44.64 3.25,45 10.4,45 v16.5,51.1
  Bottom 0.3: v23.7,55.62 21.02,55.62 v16.5,51.1
DRV_ENN_CFG6  (via drill 0.3)
  Top 0.254: TMC2100.22 34.98,51.75 35.75,50.98 v39.2,50.98
  Top 0.3: INTERFACE_TO_UC/MC.8 v21.15,23.45
  Route3 0.254: 40.4,35.8 42.5,37.9 42.5,40.5 40.34,42.66 40.34,49.84
  Route3 0.3: v39.2,50.98 40.34,49.84 40.4,49.77 | 40.4,35.8 28.05,23.45 v21.15,23.45
ERROR  (via drill 0.3)
  Top 0.254: TMC2100.20 34.48,50.75 35.25,49.98 38.3,49.98 38.6,49.67 40.5,49.67 41.9,51.08 v41.9,56.8
  Top 0.3: 2.89,61.36 INTERFACE_TO_UC/MC.37 2.9,62.3 3.4,62.8 v10.8,62.8
  Route3 0.3: v41.9,56.8 41.9,59 35.5,65.4 14.3,65.4 13.4,65.4 v10.8,62.8
EXT_DIR
  Top 0.406: R14.2 42.2,22.5 41.7,23 41.7,24.6 | 41.7,24.6 41.7,25 42.3,25.6 D3.3 | X2.1 41.7,24.6
EXT_DIR_CON
  Top 0.406: R14.1 45.6,22.5 | 45.6,22.5 R12.2 | 45.6,22.5 45.6,23.3 45.92,23.62 REF2.1
EXT_STEP
  Top 0.406: R15.2 42.1,19.6 41.7,19.2 41.7,18.4 | 41.7,18.4 41.7,17.1 42.35,16.45 D4.3 | X1.1 41.7,18.4
EXT_STEP_CON
  Top 0.406: R15.1 45.6,19.6 | 45.6,19.6 R13.2 | 45.6,19.6 45.6,20.4 46.28,21.08 REF2.2
GND  (via drill 0.3, 0.3 pad 0.3, 0.35, 3.2 pad 6.35)
  Top 0.254: 33,52.75 32.8,52.55 32.8,52.75 | 37.17,52.75 C6.2 37.06,52.75 v35.7,52.75 TMC2100.24
  Bottom 0.5: v32.8,52.5 33.05,52.75 v35.7,52.75
  other vias: 4,81 4,4 51,81 51,4 12.2,7.8 18.1,9.6 21.7,9.6 8,10 3.9,10 2.2,12.5 2.7,7.8 9.7,7.8 20.4,6 29.8,42.7 29.8,62.3 30.8,62.3 31.8,62.3 28.55,49.17 37.6,22.5 49.6,22.5 49.6,19.2 49.6,25.5 49.6,15.6 12.7,37 31.8,42.7 30.8,42.7 14.5,24.2 2.2,17.1 14.4,21.4 12.7,21.4 12.7,24.2 16.1,24.2 16.1,21.4 7.9,11.9 11.2,11.9 14.4,13.4 19.2,13.4 14.4,15.5 12.7,15.5 16.3,16.1 14.4,17.9 12.7,17.3 12.7,19.1 22.1,13.4 22.1,15.6 24.6,14.6 26,15.9 21.9,17.6 20.6,18.9 21.7,20.1 23,18.7 19.2,22.7 24.6,20.4 23.3,21.6 24.7,22.5 26.7,20.6 20.4,24.4 21.8,25.6 23.1,26.9 14.4,30.6 12.7,32.2 16.2,28.8 16.2,31.2 14.4,32.9 12.7,34.5 14.5,35.3 16.1,33.7 30.8,22.5 33.4,22.5 31.3,25.4 27.9,25.4 29.6,26.2 29.6,23.8 33.8,28.1 32.6,26.9 31.5,28.1 32.7,29.7 35.8,29.9 32.8,33.8 23.8,38.2 19.6,39 21.4,42 21.4,38.4 23.4,40.8 25.9,39.7 19.7,42 42.8,18 42.7,21 42.7,24.2 40.8,23.8 40.8,25.5 40.8,27.4 40.8,19.2 40.8,17.6 46.9,25.6 39.2,29.9 48.5,32.3 14.4,39.2 12.7,39.2 16.1,39.2 17.4,42 14.4,42 12.6,42 12.8,46.1 14.3,47.6 12.7,49.5 14.4,50.8 12.1,51.9 12.1,53.6 12.6,55.7 14.4,54.5 13,62.1 21.2,54.5 18.6,52 21.3,50.3 19.23,48.1 18.9,54.6 19.7,50.7 27.9,55.7 16.3,58.7 17.4,57.5 14.1,61 15.2,59.9 11.1,64.4 51.1,33.7 52.8,33.7 39.1,42.9 41.8,42.9 45,42.9 10,80 15,80 20,75 5,75 10,75 15,75 25,80 30,80 35,80 40,80 45,80 25,75 50,75 15,70 20,70 25,70 30,70 35,70 40,70 45,70 50,70 50,65 50,60 21.9,61.5 50,55 50,50 50,45 50,35 30,40 50,10 45,10 40,10 30,10 30,15 35,15 40,15 21.5,57.8 14.2,66.5 38.6,57.9 43.3,47.6 1.7,24.7 1.5,34.9 1.6,40 1.6,42.5 1.6,45.1 1.6,47.6 1.8,50.2 1.8,52.7 1.5,57.8 30.2,54.2 30.85,53.35 32.15,53.35 30.2,52.5 31.5,52.5 30.85,51.65 32.15,51.65 30.2,50.8 31.5,50.8 32.8,50.8 31.5,54.2 32.8,54.2 39.8,32.8
  pour Top (isolate 0.254, rank 6): 0,85 55,85 55,0 0,0
  pour Bottom (rank 6): 0,85 55,85 55,0 0,0
  pour Route2 (rank 6): 0,85 55,85 55,0 0,0
  pour Top (no thermals): 29.18,43.92 32.3,43.92 32.3,41.92 29.18,41.92
  pour Top (no thermals): 29.3,62.73 32.3,62.73 32.3,60.42 29.3,60.42
ID_CH1
  Top 0.3: IC1.5 26.12,5.62 28.4,7.9 28.4,12.2 18.4,22.2 3.4,22.2 2.89,22.71 INTERFACE_TO_UC/MC.7
ID_CLK  (via drill 0.3)
  Top 0.3: R1.1 v16.3,7.5 16.88,6.92 IC1.2 | INTERFACE_TO_UC/MC.4 v10.97,18.37
  Route3 0.3: v16.3,7.5 16.3,14.8 12.73,18.37 v10.97,18.37
INDEX  (via drill 0.3)
  Top 0.254: TMC2100.21 34.73,51.25 35.5,50.48 38.6,50.48 38.9,50.17 40.1,50.17 41,51.08 v41,56
  Top 0.3: INTERFACE_TO_UC/MC.38 v11.25,61.55
  Route3 0.3: v41,56 41,57.3 34.6,63.7 13.4,63.7 v11.25,61.55
INT_DIR
  Top 0.3: INTERFACE_TO_UC/MC.18 12.55,36.15 24.1,24.6 X2.3
INT_STEP
  Top 0.254: INTERFACE_TO_UC/MC.17 4.14,34.9
  Top 0.3: 4.14,34.9 11.2,34.9 27.7,18.4 X1.3
M1A  (via drill 0.3)
  Bottom 3: 39.8,53.75 MOTOR1.3
  other vias: 29.24,58.21 29.24,57.24
  pour Top (rank 2, no thermals): 30.8,55.11 30.8,56.92 29.74,56.92 29.74,58.64 28.86,58.64 28.86,56.99 29.74,56.17 30.68,56.17 30.68,55.11
  pour Bottom: 39.8,55.12 38.49,55.12 arc-41 37.83,55.37 36.77,56.31 arc41 35.45,56.8 31.5,56.8 arc-90 30.5,57.8 30.5,58 arc90 29.5,59 arc90 28.5,58 28.5,55.5 arc90 29,55 33.87,55 arc-45 35.29,54.41 36.67,53.03 arc44 38.03,52.45 39.8,52.4
M1A2  (via drill 0.3)
  Bottom 3: 37.9,61.1 41.85,61.1 arc-90 MOTOR1.4
  other vias: 32.42,58.61 32.42,57.69
  pour Top (rank 2, no thermals): 31.68,55.11 31.68,57.55 31.86,57.55 31.86,59.3 32.92,59.3 32.92,56.8 31.99,55.8 31.99,55.11
  pour Bottom: 38.1,59.75 34.1,59.75 arc90 33.1,58.75 33.1,58.3 arc-90 32.1,57.3 32,57.3 arc-90 31,58.3 31,59.2 arc-90 34.1,62.45 38.1,62.45
M1B1  (via drill 0.3)
  Bottom 3: MOTOR1.1 45.68,46.73 arc-45 41.99,45.2 40.3,45.2
  other vias: 29.11,47.42 29.11,46.5
  pour Top (no thermals): 30.8,49.8 30.8,47.92 29.8,47.92 29.8,45.99 28.68,45.99 28.68,47.8 29.8,48.92 30.68,48.92 30.68,49.8
  pour Bottom: 33.15,45.5 31.4,45.5 arc-90 30.4,46.5 30.4,47.3 arc90 29.4,48.3 arc90 28.4,47.3 28.4,44.84 arc90 29.4,43.84 41.7,43.84 41.73,46.55 34.83,46.55 arc46 34.1,46.24 33.57,45.68 arc-46
M1B2  (via drill 0.3)
  Bottom 3: MOTOR1.2 43.5,50.25 arc45 42.26,49.74 arc-45 39.94,48.77 33.69,48.77 v32.3,47.39
  other vias: 32.3,46.46
  pour Top (rank 2, no thermals): 31.74,49.8 31.74,45.85 32.8,45.85 32.8,48.05 31.86,48.8 31.86,49.8
N$1
  Top 0.3: C3.1 14.2,8.2 16.12,6.28 IC1.3 19.38,6.28 19.9,6.8 R2.2
N$2
  Top 0.3: R_ID.1 24.5,7.6 23.82,6.92 | IC1.7 23.82,6.92 | C_ID.1 26.6,7.7 25.82,6.92 23.82,6.92
N$3
  Top 0.254: R_SPI.2 25.2,47 28.45,50.25 TMC2100.10
N$4
  pour Bottom (isolate 0.1): 33.2,53.05 35.7,53.05 arc-90 36,52.75 arc-90 35.7,52.45 33.2,52.45
  pour Route3 (isolate 0.1): 35.7,53.05 arc-90 36,52.75 arc-90 35.7,52.45 arc-90 35.4,52.75 arc-90
  pour Route2 (isolate 0.1): 35.7,53.05 arc-90 36,52.75 arc-90 35.7,52.45 arc-90 35.4,52.75 arc-90
N$5
  Top 0.254: R_SD.2 26.5,49.1 28.15,50.75 TMC2100.9
N$7
  Top 0.254: TMC2100.25 35.12,53.25 36.21,54.34 C6.1 38.14,54.34 38.3,54.17 38.3,52.92 38.55,52.67 39.33,52.67 R6.1
N$8
  Top 0.254: TMC2100.28 34.31,54.75 34.67,55.11 34.67,55.86 35.55,56.74 C8.1
N$9
  Top 0.254: TMC2100.27 34.62,54.25 35.3,54.92 35.3,55.42 35.77,55.9 37.77,55.9 38.05,56.17 38.05,56.71 C8.2
N$10
  Top 0.254: TMC2100.29 33.25,55.75 33.55,56.05 33.92,56.05 35.49,57.61 36.49,57.61 36.67,57.8 36.67,58.67 36.8,58.8 C7.2 37.34,58.67
N$11
  Top 0.254: TMC2100.26 34.88,53.75 36.05,54.92 36.05,55.17 36.26,55.39 39.36,55.39 | C9.2 39.8,55.83 39.36,55.39 | 39.36,55.39 R6.2
N$14
  Top 0.3: R17.2 42.9,31 43.15,30.75 R10.1 C14.2
SENSEA
  Top 0.254: TMC2100.33 31.25,56.75 30.8,57.2 R5.2
  Top 0.3: RSENSE_A.1 30.5,59.5 30.8,59.2 R5.2
  Bottom 0.3: RSENSE_A.1 18.34,59.5 15.67,56.83 13.84,55 13.54,54.7 TEST_POINT2.P$1
SENSEB  (via drill 0.3)
  Top 0.3: TMC2100.14 31.25,48.25 30.8,47.8 R7.2 30.8,46 30.3,45.5 RSENSE_B.1 v19.7,45.5
  Bottom 0.3: TEST_POINT3.P$1 15.3,4.78 15.3,41.1 v19.7,45.5
  pour Top (rank 3, no thermals): 30.18,46.3 31.43,46.3 31.18,47.17 30.18,47.17
UNUSED
  Top 0.254: TMC2100.17 32.75,49.02 33.3,48.48 37.45,48.48 37.75,48.17 41.27,48.17 44,50.9 44,58.1 36.1,66 18,66 11.01,59.01 INTERFACE_TO_UC/MC.36
VCC_IO  (via drill 0.3)
  Top 0.254: C5.1 v27.2,50.9 27.55,51.25 TMC2100.8
  Top 0.3: R8.1 R9.2
  Top 0.5: D4.2 47.1,17.4 47.6,16.9 53,16.9 53.7,17.6 53.7,25.6 v52.75,26.55 D3.2 | R9.2 v19.32,16.32
  Route3 0.5: v19.32,16.32 24.5,21.5 v40.8,21.5
  Bottom 0.5: v52.75,26.55 41.8,26.55 | 41.8,26.55 37.75,26.55 24.8,39.5 24.8,48.5 v27.2,50.9 | v40.8,21.5 41.8,22.5 41.8,26.55
VM  (via drill 0.3, 0.35)
  Top 0.3: v35.8,38.33 35.8,38 35.17,38 C11.1
  Top 1: INTERFACE_TO_UC/MC.1 v2.89,14.71 | v2.89,14.71 v2.9,14.7 2.9,14.2 v2.1,14.2 | v2.89,14.71 v2.89,13.71 v2.9,13.7
  Top 1.9: PWR.2 38.3,74.7 D1.C
  Top 2.75: C12.+ 35.17,38
  Top 3: C13.+ v41.7,66
  other vias: 33.86,58.41 33.86,57.49 35.88,42.8 36.84,42.8 42.3,65.2 42.3,66.8 37,38.33 36.4,37.52
  pour Route3 (isolate 0.1, rank 5): 0,85 55,85 55,0 0,0
  pour Top (no thermals): 32.24,49.8 32.24,48.61 34.05,46.86 34.05,45.74 35.4,45.74 35.4,42.08 37.3,42.08 37.3,49.8
  pour Top (no thermals): 32.24,55.11 32.92,55.11 32.92,55.61 35.3,57.86 35.3,59.3 33.24,59.3 33.24,56.67 32.24,55.67

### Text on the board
Top: Top
Route2: Inner1
Route3: Inner2
Bottom: Bottom
tPlace: 7..46V | GND | +VM | GND | A2 | Silkscreen Top | A1 | B2 | B1 | GND | GND | DIR | DIR | INT | EXT | STEP | GND | STEP | GND | S/D | TMC2100-EVAL v1.3
bPlace: TMC-Evaluation-Platform: | TMC2100-Eval | Silkscreen Bottom | Interfaces: | S/D | Voltage: | 7..46V | Phase current: | 1.2A RMS | v1.3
